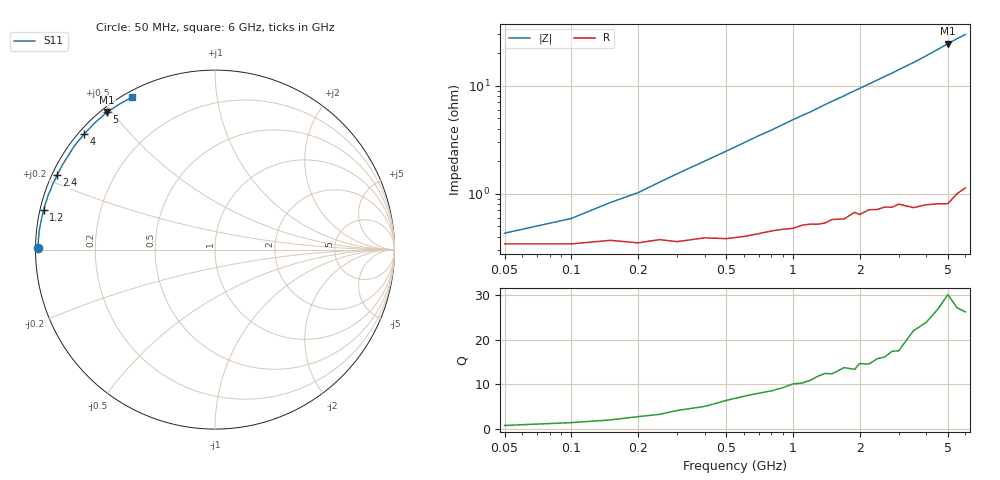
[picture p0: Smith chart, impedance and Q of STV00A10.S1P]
! SIEMENS Discrete & RF Semiconductors
! BA892
! Si PIN Diode in SCD-80
! IF = 100 mA
! S-Parameters:  September  1997
# GHz  S  MA  R  50
!  f  S11
! GHz  MAG  ANG
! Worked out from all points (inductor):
!   34 points, 50 MHz to 6 GHz, reference 50 ohm
!   read as one part to ground: L = 782 pH near 250 MHz
!   highest Q = 27.1 at 5 GHz (marker M1), where L = 774 pH
!   S11 on the Smith chart (normalised r, x): 50 MHz: 0.01, +0.01; 1.2 GHz: 0.01, +0.11; 2.4 GHz: 0.01, +0.22; 4 GHz: 0.02, +0.38; 5 GHz: 0.02, +0.49; 6 GHz: 0.02, +0.59
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0.05  0.9864 179.4
0.1  0.9863 178.9
0.15  0.9853 178.3
0.2  0.9861 177.8
0.25  0.9851 177.2
0.3  0.9857 176.6
0.5  0.9848 174.4
0.7  0.9831 172.2
0.8  0.9822 171.2
1  0.9812 169.0
1.2  0.9796 167.0
1.4  0.9791 164.8
1.6  0.9776 162.8
1.7  0.9775 161.8
1.8  0.9759 160.7
1.9  0.9743 159.7
2  0.9755 158.7
2.2  0.9731 156.7
2.4  0.9732 154.7
2.6  0.9719 152.7
2.8  0.9723 150.8
3  0.9707 148.7
3.5  0.9735 143.8
4  0.9727 138.6
4.5  0.9732 133.3
5  0.9742 128.1
5.5  0.9696 123.0
6  0.967 118.6
